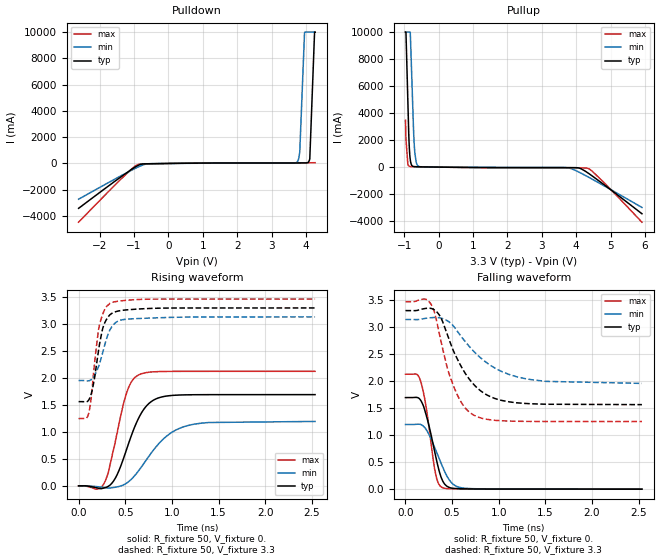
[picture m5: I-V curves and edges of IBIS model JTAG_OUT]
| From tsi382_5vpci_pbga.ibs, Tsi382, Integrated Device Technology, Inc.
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|   MODEL JTAG_OUT
[Model]   JTAG_OUT
Model_type  Output
C_comp 1.649p 1.575p 1.712p
Polarity   Non-Inverting
Enable   Active-High
Vmeas =   1.65V
|   typ   min   max
[Model Spec]
[Temperature Range]   25   125   -40
[Voltage Range] 3.3 3.135 3.465
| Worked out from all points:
|   slope of the pulldown table from 0 to 0.495 V, typ, clamps not added: 28.2 ohm
|   slope of the pullup table from 0 to 0.495 V, typ, clamps not added: 32.8 ohm
|   rising waveform, R_fixture 50, V_fixture 0.: 20-80 % time 229ps typ, 344ps min, 168ps max; typ from 0 V to 1.69 V
|   rising waveform, R_fixture 50, V_fixture 3.3: 20-80 % time 103ps typ, 130ps min, 90ps max; typ from 1.56 V to 3.3 V
|   falling waveform, R_fixture 50, V_fixture 0.: 20-80 % time 136ps typ, 179ps min, 106ps max; typ from 1.69 V to 0 V
|   falling waveform, R_fixture 50, V_fixture 3.3: 20-80 % time 317ps typ, 447ps min, 225ps max; typ from 3.3 V to 1.56 V
[Pulldown]
-2.613V   -3.415A    -2.72A     -4.469A
-1.41V    -1.072A    -979.5mA   -1.262A
-868mV    -126.7mA   -251.3mA   -64.57mA
-534.3mV  -20.83mA   -16.62mA   -27.15mA
3.727V    37.09mA    88.44mA    50.52mA
3.776V    37.18mA    283.1mA    50.59mA
3.818V    37.33mA    860.9mA    50.65mA
3.957V    39.38mA    9.949A     51.13mA
4.061V    88.7mA     10A        52.38mA
4.11V     353.8mA    10A        53.29mA
4.249V    10A        10A        57.48mA
4.263V    10A        10A        58.61mA
[Pullup]
-962.7mV  10A        10A        3.476A
-948.8mV  10A        10A        2.071A
-893.2mV  4.867A     10A        202.9mA
-858.4mV  1.841A     10A        71.37mA
-823.7mV  557.1mA    10A        45.9mA
-761.1mV  77.1mA     5.268A     37.55mA
-719.4mV  36.46mA    2.228A     35.04mA
-691.6mV  28.89mA    1.08A      33.5mA
-580.3mV  21.11mA    59.76mA    27.6mA
3.688V    -38.12mA   -32.97mA   -52.41mA
4.328V    -406.9mA   -701.1mA   -83.52mA
5.913V    -3.455A    -2.989A    -4.08A
[Ramp]
dV/dt_r 1.015/228.756p .717/344.077p 1.275/168.409p
dV/dt_f 1.043/317.593p .709/447.763p 1.33/225.281p
[Rising Waveform]
R_fixture = 50
V_fixture = 0.
0s        714nV      0V         582.7nV
270ps     -41.37mV   -28.72mV   36.89mV
325ps     -582.9uV   -39.73mV   288.4mV
390ps     132mV      -26.27mV   790.9mV
505ps     628mV      40.6mV     1.671V
565ps     928.7mV    122.6mV    1.927V
645ps     1.261V     284.1mV    2.059V
815ps     1.601V     691.3mV    2.116V
1.155ns   1.688V     1.111V     2.124V
2.535ns   1.692V     1.195V     2.125V
[Rising Waveform]
R_fixture = 50
V_fixture = 3.3
V_fixture_min = 3.135
V_fixture_max = 3.465
0s        1.562V     1.954V     1.249V
110ps     1.596V     1.949V     1.355V
135ps     1.703V     1.97V      1.627V
165ps     1.94V      2.03V      2.169V
215ps     2.523V     2.219V     2.907V
270ps     2.981V     2.548V     3.235V
345ps     3.186V     2.92V      3.393V
435ps     3.247V     3.066V     3.428V
575ps     3.272V     3.099V     3.45V
2.535ns   3.3V       3.135V     3.465V
[Falling Waveform]
R_fixture = 50
V_fixture = 0.
0s        1.692V     1.195V     2.125V
120ps     1.695V     1.199V     2.122V
165ps     1.636V     1.194V     1.983V
215ps     1.411V     1.118V     1.585V
315ps     678.9mV    762.5mV    350.5mV
350ps     411.9mV    613.4mV    119.8mV
395ps     167.6mV    425.2mV    29.01mV
490ps     21.57mV    126mV      8.027mV
630ps     6.368mV    18.7mV     3.312mV
2.535ns   12.24uV    11.96uV    22.03uV
[Falling Waveform]
R_fixture = 50
V_fixture = 3.3
V_fixture_min = 3.135
V_fixture_max = 3.465
0s        3.3V       3.135V     3.465V
275ps     3.339V     3.169V     3.415V
315ps     3.306V     3.172V     3.247V
380ps     3.168V     3.161V     2.738V
520ps     2.532V     3.002V     1.887V
630ps     2.171V     2.75V      1.524V
750ps     1.903V     2.515V     1.352V
960ps     1.675V     2.237V     1.272V
1.27ns    1.585V     2.047V     1.253V
2.535ns   1.562V     1.955V     1.249V
